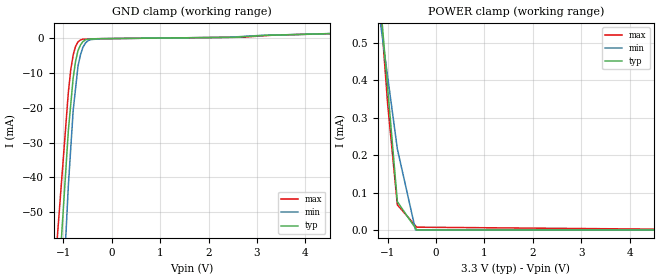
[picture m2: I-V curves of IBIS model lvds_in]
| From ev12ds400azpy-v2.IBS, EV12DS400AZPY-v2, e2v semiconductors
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[Model] lvds_in
Model_type Input
Vinl = 1.15000V
Vinh = 1.35000V
C_comp 559.000fF 532.000fF 586.000fF
| variable typ   min   max
[Voltage Range] 3.30000V 3.15000V 3.45000V
[POWER Clamp Reference] 3.30000V 3.15000V 3.45000V
[GND Clamp Reference] 0.00000V 0.00000V 0.00000V
[Temperature Range]   25   110   -40
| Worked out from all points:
|   GND clamp passes 1 mA (typ) near -0.59 V on its own axis
[GND Clamp]
-3.3V     -545.2mA   -713.2mA   -453.1mA
-900mV    -26.66mA   -42.42mA   -15.61mA
-850mV    -19.06mA   -31.62mA   -9.137mA
-800mV    -11.45mA   -20.82mA   -4.872mA
-750mV    -6.644mA   -14.43mA   -2.374mA
-700mV    -3.644mA   -8.033mA   -1.13mA
-650mV    -2.043mA   -4.891mA   -594.5uA
-600mV    -1.066mA   -2.738mA   -344.2uA
-500mV    -350.1uA   -848uA     -300.8uA
-225mV    -201.7uA   -218.8uA   -203.4uA
2.7V      333.1uA    427.9uA    211.7uA
6.6V      2.046mA    2.014mA    1.992mA
[POWER Clamp]
-3.3V     3.862mA    2.621mA    4.333mA
-1V       378.4uA    408.7uA    335.3uA
-800mV    75.47uA    216.4uA    67.09uA
-500mV    18.87uA    43.28uA    22.36uA
-425mV    4.717uA    0A         11.18uA
-400mV    0A         0A         7.455uA
6.6V      0A         0A         0A
